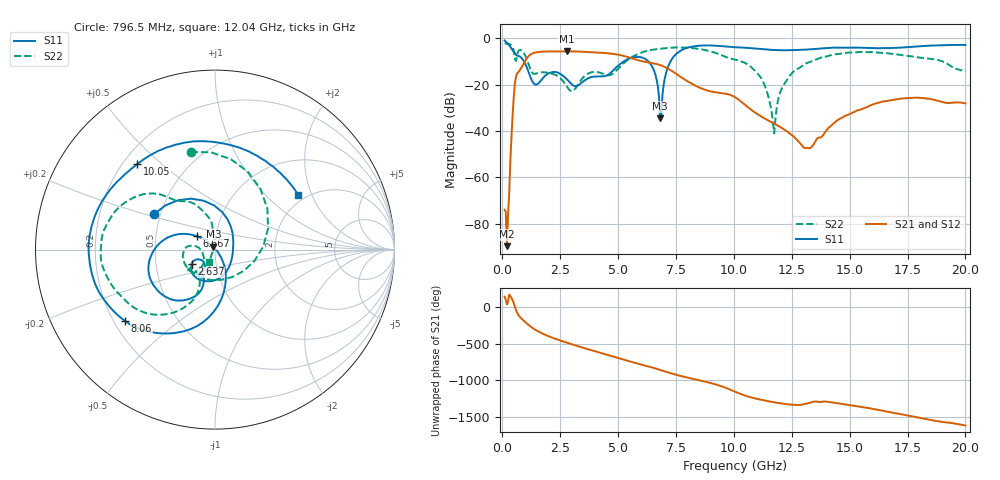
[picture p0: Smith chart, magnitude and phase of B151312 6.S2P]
!  2-Port S-parameters saved by WinCal
! VAR MeasName=S-Parameters (CALIBRATED_DATA) read from VNA (N5244A)
! VAR MeasDate=12/8/2015 5:44:11 PM
! VAR NAME=B151312 6
! VAR FILENAME=B151312 6.S2P
! VAR DATE=12/8/2015 5:44:11 PM
! VAR PHYS_PORTS=1,2
# Hz S DB R 50
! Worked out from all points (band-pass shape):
!   401 points, 100 MHz to 20 GHz, reference 50 ohm
!   highest |S21| = -5.63 dB at 2.787 GHz (marker M1); lowest = -89.7 dB at 199.5 MHz (marker M2)
!   |S21| within 3 dB of the highest: 1.057 GHz to 5.605 GHz (4.547 GHz wide, 137 % of centre)
!   lowest |S11| = -34.6 dB at 6.816 GHz (marker M3), VSWR 1.04, Z = 49.1 + j1.61 ohm
!   |S11| at or under -10 dB: 939.6 MHz to 5.239 GHz (4.299 GHz wide, 139 % of centre); 6.313 GHz to 7.261 GHz (948.4 MHz wide, 14 % of centre)
!   |S22| runs from -41.0 to -2.2 dB; largest |S21 - S12| = 0.0013
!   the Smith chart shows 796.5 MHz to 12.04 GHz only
!   S11 on the Smith chart (normalised r, x): 796.5 MHz: 0.46, +0.22; 2.637 GHz: 0.76, -0.13; 6.667 GHz: 0.81, +0.12; 8.06 GHz: 0.24, -0.33; 10.05 GHz: 0.26, +0.42; 12.04 GHz: 1.81, +1.60
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1e8  -0.91 -41.9  -73.91 141.1  -74.63 150.3  -2.19 169.3
1.995e8  -1.91 -77.0  -89.68 36.3  -85.90 74.7  -2.28 158.2
5.4775e8  -6.41 -166.5  -19.28 2.5  -19.27 2.5  -9.10 107.0
7.965e8  -8.14 149.6  -13.14 -147.1  -13.14 -147.2  -5.03 103.9
1.294e9  -18.50 32.0  -6.55 77.6  -6.55 77.6  -14.85 -57.4
1.74175e9  -17.27 -61.9  -5.74 -2.7  -5.74 -2.7  -14.61 -157.1
2.63725e9  -16.30 -148.1  -5.63 -110.7  -5.63 -110.7  -18.66 170.0
2.7865e9  -17.59 -152.3  -5.63 -126.1  -5.63 -126.1  -20.74 172.8
3.43325e9  -19.09 -120.5  -5.77 170.2  -5.77 170.2  -17.54 -128.1
5.075e9  -11.22 -112.2  -7.19 17.0  -7.19 17.1  -12.36 -112.4
6.667e9  -17.90 143.6  -11.07 -122.7  -11.08 -122.7  -4.70 -153.0
6.7665e9  -25.07 132.6  -11.35 -132.5  -11.36 -132.5  -4.57 -155.6
6.81625e9  -34.57 118.9  -11.50 -137.5  -11.52 -137.5  -4.51 -157.0
7.264e9  -9.95 -87.6  -13.71 178.4  -13.69 178.4  -4.06 -168.4
8.06e9  -3.88 -141.7  -18.86 113.6  -18.86 113.4  -4.05 169.7
1.005e10  -3.82 132.3  -25.39 -74.9  -25.41 -75.1  -9.15 128.5
1.11445e10  -4.60 81.3  -33.50 177.3  -33.56 177.4  -16.62 96.8
1.169175e10  -5.01 52.5  -36.51 143.4  -36.59 143.4  -36.79 108.8
1.204e10  -5.12 33.5  -38.45 125.5  -38.48 125.9  -22.20 -114.9
1.338325e10  -4.68 -32.1  -46.51 143.6  -46.52 143.6  -9.88 -141.6
1.67165e10  -4.20 -111.8  -26.86 7.9  -26.67 7.8  -6.53 154.0
2e10  -2.86 -147.6  -28.06 -175.5  -28.06 -176.7  -13.89 129.9
